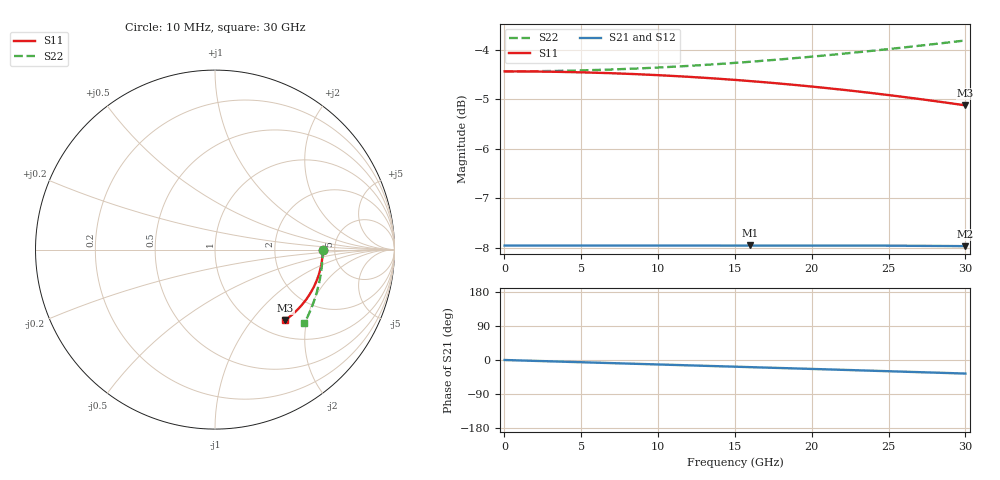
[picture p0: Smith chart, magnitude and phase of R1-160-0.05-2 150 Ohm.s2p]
!version-1
!date-04.2021
# GHz S RI R 50
!Freq ReS11 ImS11 ReS21 ImS21 ReS12 ImS12 ReS22 ImS22
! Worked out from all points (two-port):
!   601 points, 10 MHz to 30 GHz, reference 50 ohm
!   highest |S21| = -7.96 dB at 16.01 GHz (marker M1); lowest = -8.0 dB at 30 GHz (marker M2)
!   |S21| within 3 dB of the highest: start of sweep to end of sweep
!   lowest |S11| = -5.1 dB at 30 GHz (marker M3), VSWR 3.49, Z = 65.9 - j74.8 ohm
!   |S11| at or under -10 dB: nowhere
!   |S22| runs from -4.4 to -3.8 dB; largest |S21 - S12| = 1.4e-15
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0.01  0.6 -0.000144  0.4 -8.13e-05  0.4 -8.13e-05  0.6 -0.000144
0.16  0.6 -0.0023  0.4 -0.0013  0.4 -0.0013  0.6 -0.0023
2.51  0.5986 -0.0361  0.3995 -0.0204  0.3995 -0.0204  0.5993 -0.0361
5.01  0.5943 -0.0719  0.3979 -0.0407  0.3979 -0.0407  0.597 -0.072
7.51  0.5873 -0.1075  0.3954 -0.0609  0.3954 -0.0609  0.5934 -0.1077
8.76  0.5827 -0.1252  0.3937 -0.071  0.3937 -0.071  0.591 -0.1255
10.01  0.5773 -0.1428  0.3918 -0.081  0.3918 -0.081  0.5882 -0.1432
11.26  0.5713 -0.1602  0.3896 -0.091  0.3896 -0.091  0.5851 -0.1608
12.51  0.5645 -0.1775  0.3871 -0.101  0.3871 -0.101  0.5817 -0.1783
13.76  0.557 -0.1947  0.3844 -0.1109  0.3844 -0.1109  0.5778 -0.1958
15.01  0.5488 -0.2117  0.3814 -0.1208  0.3814 -0.1208  0.5737 -0.2131
16.01  0.5417 -0.2251  0.3788 -0.1287  0.3788 -0.1287  0.5701 -0.2269
18.01  0.526 -0.2516  0.3731 -0.1444  0.3731 -0.1444  0.5623 -0.2543
20.01  0.5084 -0.2774  0.3668 -0.1598  0.3668 -0.1598  0.5536 -0.2813
21.26  0.4964 -0.2932  0.3624 -0.1694  0.3624 -0.1694  0.5477 -0.298
22.51  0.4837 -0.3087  0.3578 -0.1789  0.3578 -0.1789  0.5415 -0.3145
23.76  0.4701 -0.3238  0.3529 -0.1883  0.3529 -0.1883  0.535 -0.3309
25.01  0.4558 -0.3385  0.3477 -0.1976  0.3477 -0.1976  0.5281 -0.3471
27.26  0.4281 -0.364  0.3376 -0.214  0.3376 -0.214  0.515 -0.3757
29.06  0.4042 -0.3833  0.3288 -0.2269  0.3288 -0.2269  0.5039 -0.3982
29.86  0.393 -0.3916  0.3247 -0.2326  0.3247 -0.2326  0.4987 -0.4081
30  0.391 -0.393  0.324 -0.2335  0.324 -0.2335  0.4978 -0.4098
